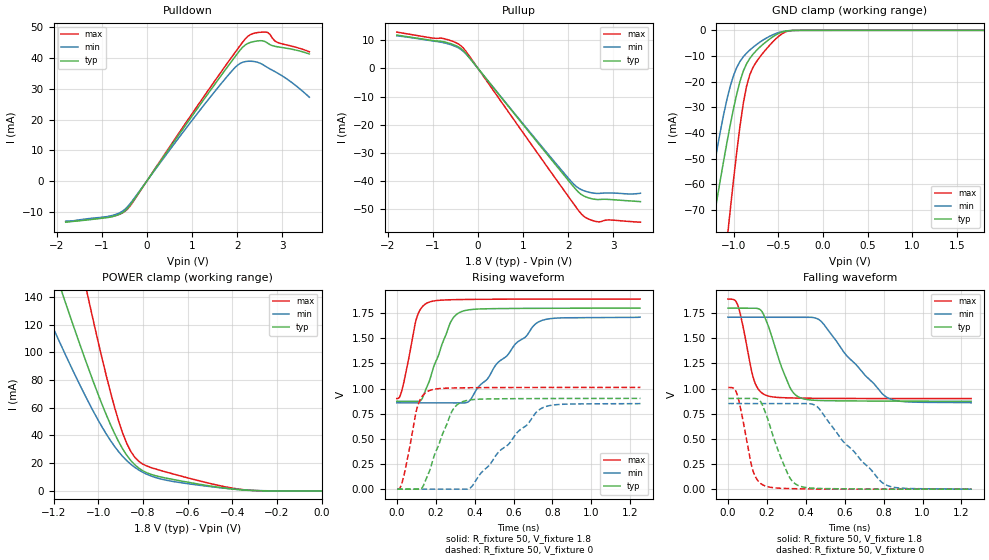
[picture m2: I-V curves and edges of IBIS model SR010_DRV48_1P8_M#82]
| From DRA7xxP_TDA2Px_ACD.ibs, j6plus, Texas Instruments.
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| Model based on original model for DDR_SEIOPB_V
|   Sub model SR010_DRV48_1P8
[model]   SR010_DRV48_1P8_M#82
|[Description]  [1.8V-I/O-X-X]
|   , ,
|[Input Load]
|[Output Drive]
|Voltage   1.8V
|Mode   I/O
Model_type   I/O
Polarity   Non-Inverting
Enable   Active-Low
Vinl =  0.775
Vinh =  1.025
Cref =  15.0000pF
Rref =  100.0000M
Vref =  0V
Vmeas =  0.9
C_comp   2p   2p   2p
[Model Spec]
Vinl   0.78   0.735   0.825
Vinh   1.02   0.975   1.065
[Receiver Thresholds]
Tslew_ac = 0.5n
Vth = 0.9
Vth_max = 0.945
Vth_min = 0.81
Vinh_ac = 0.2
Vinh_dc = 0.125
Vinl_ac = -0.2
Vinl_dc = -0.125
[Temperature Range]   25   125   -40
[Voltage Range]   1.8   1.71   1.89
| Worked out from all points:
|   slope of the pulldown table from 0 to 0.27 V, typ, clamps not added: 46.9 ohm
|   slope of the pullup table from 0 to 0.27 V, typ, clamps not added: 49.7 ohm
|   GND clamp passes 1 mA (typ) near -0.48 V on its own axis
|   POWER clamp passes 1 mA (typ) near -0.38 V on its own axis
|   rising waveform, R_fixture 50, V_fixture 1.8: 20-80 % time 102ps typ, 248ps min, 60.4ps max; typ from 0.874 V to 1.8 V
|   rising waveform, R_fixture 50, V_fixture 0: 20-80 % time 103ps typ, 249ps min, 60.4ps max; typ from 0 V to 0.903 V
|   falling waveform, R_fixture 50, V_fixture 1.8: 20-80 % time 98.7ps typ, 228ps min, 62.4ps max; typ from 1.8 V to 0.874 V
|   falling waveform, R_fixture 50, V_fixture 0: 20-80 % time 101ps typ, 233ps min, 61.7ps max; typ from 0.903 V to 0 V
[POWER_clamp]
-1.8V     464.6mA    344.4mA    740.8mA
-1.273V   197mA      143.3mA    314.4mA
-1.164V   144mA      104.2mA    229mA
-1.145V   135.3mA    97.86mA    215mA
-1.055V   93.25mA    67.59mA    146.5mA
-1.036V   85.18mA    61.89mA    133.3mA
-909.1mV  35.72mA    28.41mA    50.73mA
-872.7mV  25.87mA    21.94mA    34.5mA
-818.2mV  16.45mA    15.08mA    21.33mA
-690.9mV  9.084mA    7.592mA    13.42mA
-400mV    1.38mA     1.43mA     2.039mA
0V        227.3nA    761nA      1.176uA
[Pulldown]
-1.8V     -13.45mA   -13.11mA   -13.3mA
-818.2mV  -11.81mA   -11.44mA   -11.72mA
-600mV    -10.83mA   -10.36mA   -10.81mA
-436.4mV  -9.068mA   -8.512mA   -9.288mA
1.255V    26.38mA    24.53mA    27.32mA
1.855V    38.53mA    35.35mA    39.84mA
2.073V    42.76mA    38.34mA    44.25mA
2.291V    45.11mA    39mA       47.65mA
2.618V    45.4mA     37.45mA    48.49mA
2.727V    44.4mA     36.48mA    47.76mA
2.891V    43.71mA    35.16mA    45.15mA
3.6V      41.36mA    27.26mA    42.08mA
[Pullup]
-1.8V     11.9mA     11.66mA    12.97mA
-1.036V   10.04mA    9.888mA    10.91mA
-763.6mV  9.523mA    9.186mA    10.68mA
-490.9mV  8.144mA    7.787mA    9.204mA
-327.3mV  6.377mA    6.133mA    7.311mA
2.018V    -40.23mA   -39.43mA   -46mA
2.182V    -43.37mA   -42.12mA   -49.65mA
2.345V    -45.48mA   -43.6mA    -52.72mA
2.509V    -46.4mA    -44.3mA    -54.07mA
2.673V    -46.74mA   -44.55mA   -54.7mA
2.891V    -46.69mA   -44.38mA   -54.01mA
3.6V      -47.48mA   -44.49mA   -54.81mA
[GND_clamp]
-1.8V     -200.8mA   -187.9mA   -345.9mA
-1.327V   -95.75mA   -76.22mA   -171.1mA
-1.255V   -80.19mA   -60.47mA   -144.9mA
-1.218V   -72.53mA   -52.92mA   -131.9mA
-1.073V   -43.32mA   -26.59mA   -81.54mA
-1.036V   -36.61mA   -21.6mA    -69.55mA
-963.6mV  -24.61mA   -14.37mA   -47.01mA
-854.5mV  -12.98mA   -8.864mA   -21.66mA
-781.8mV  -9.263mA   -6.573mA   -14.36mA
-672.7mV  -5.498mA   -3.827mA   -8.897mA
-345.5mV  -48.81uA   -73.08uA   -79.37uA
1.8V      227.3nA    3.986uA    988nA
[Ramp]
dV/dt_f 0.55607755/98.772336p 0.51146085/0.22854408n 0.59373026/62.375299p
dV/dt_r 0.54247628/0.10339817n 0.51203339/0.24919779n 0.60759687/60.428298p
R_load = 50
[Rising Waveform]
R_fixture = 50
V_fixture = 1.8
V_fixture_min = 1.71
V_fixture_max = 1.89
0s        873.8mV    858.6mV    900.8mV
32.29ps   873.2mV    858.6mV    1.03V
103.6ps   872.5mV    858.6mV    1.712V
162.7ps   1.051V     858.6mV    1.857V
275ps     1.655V     858.4mV    1.883V
335.1ps   1.767V     857mV      1.886V
374.4ps   1.784V     879.5mV    1.887V
513.2ps   1.795V     1.245V     1.889V
732.2ps   1.798V     1.667V     1.89V
1.25ns    1.8V       1.71V      1.89V
[Rising Waveform]
R_fixture = 50
V_fixture = 0
V_fixture_min = 0
V_fixture_max = 0
2.062ps   0V         0V         0V
35.8ps    0V         0V         128.6mV
108.1ps   0V         0V         832mV
132.2ps   19.8mV     0V         928.3mV
165.8ps   169.5mV    0V         979mV
279.9ps   761.3mV    0V         1.006V
340.7ps   872.1mV    0V         1.008V
383.5ps   889.1mV    22.6mV     1.009V
746.8ps   901.1mV    807.1mV    1.011V
1.252ns   902.5mV    851.6mV    1.011V
[Falling Waveform]
R_fixture = 50
V_fixture = 1.8
V_fixture_min = 1.71
V_fixture_max = 1.89
0s        1.8V       1.71V      1.89V
49.44ps   1.8V       1.71V      1.835V
132.6ps   1.801V     1.71V      1.093V
195.5ps   1.682V     1.71V      933.5mV
313.4ps   1.033V     1.71V      907.5mV
374.5ps   906.6mV    1.71V      905.1mV
477.9ps   881.2mV    1.671V     903mV
609ps     877.5mV    1.331V     901.7mV
823.4ps   875.3mV    905.8mV    901mV
1.25ns    873.8mV    858.6mV    900.8mV
[Falling Waveform]
R_fixture = 50
V_fixture = 0
V_fixture_min = 0
V_fixture_max = 0
2.062ps   902.5mV    851.6mV    1.011V
45.14ps   902.7mV    851.6mV    954mV
126.6ps   902.7mV    851.6mV    197.5mV
188.3ps   783.8mV    851.6mV    33.95mV
306.1ps   158.5mV    851.5mV    6.257mV
366.5ps   32.31mV    851.6mV    3.696mV
461.1ps   7.505mV    815.8mV    0V
592ps     3.324mV    475.1mV    0V
810.6ps   0V         43.51mV    0V
1.252ns   0V         0V         0V
